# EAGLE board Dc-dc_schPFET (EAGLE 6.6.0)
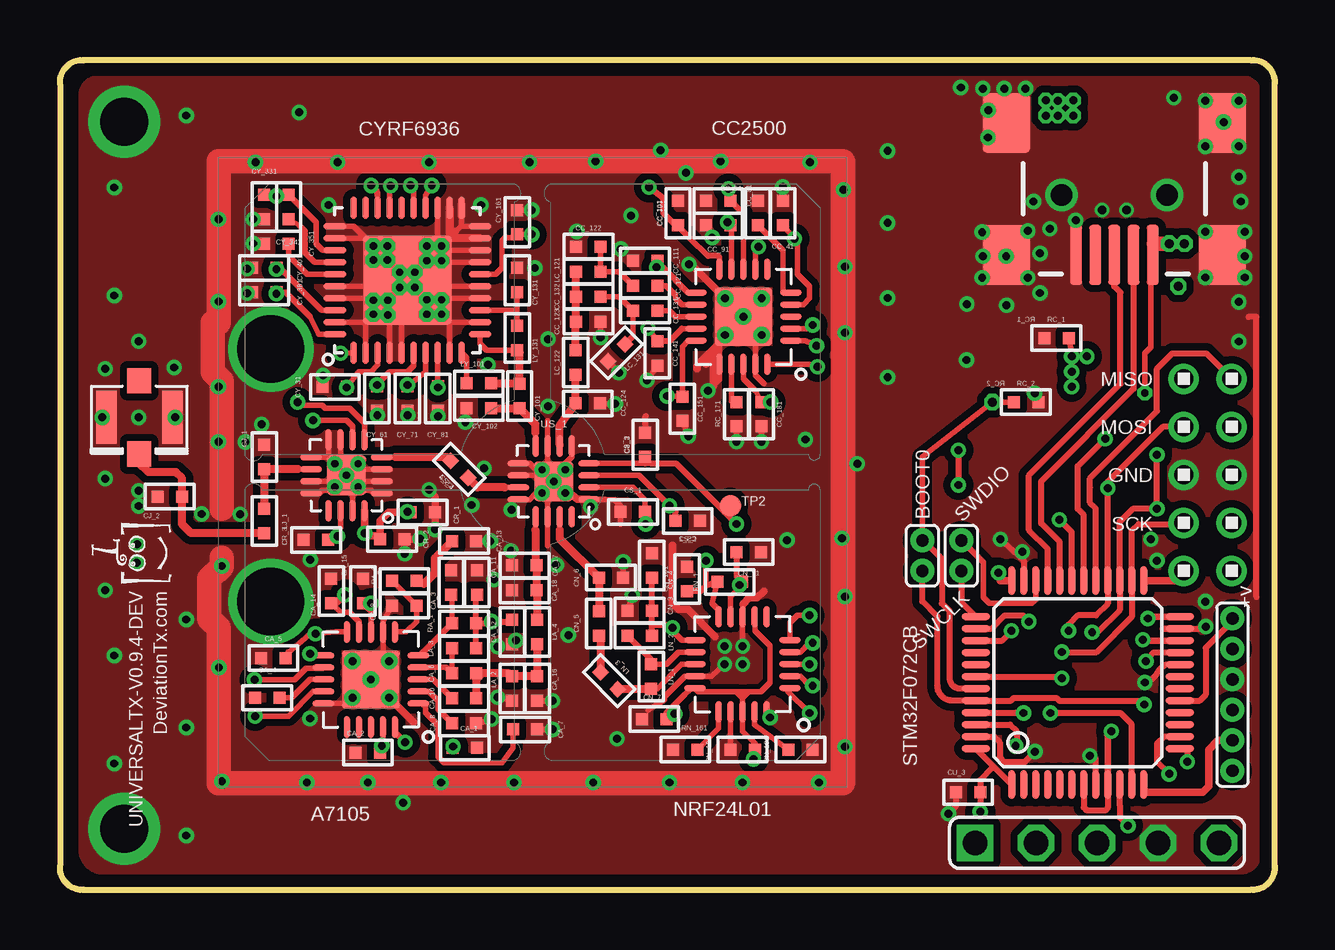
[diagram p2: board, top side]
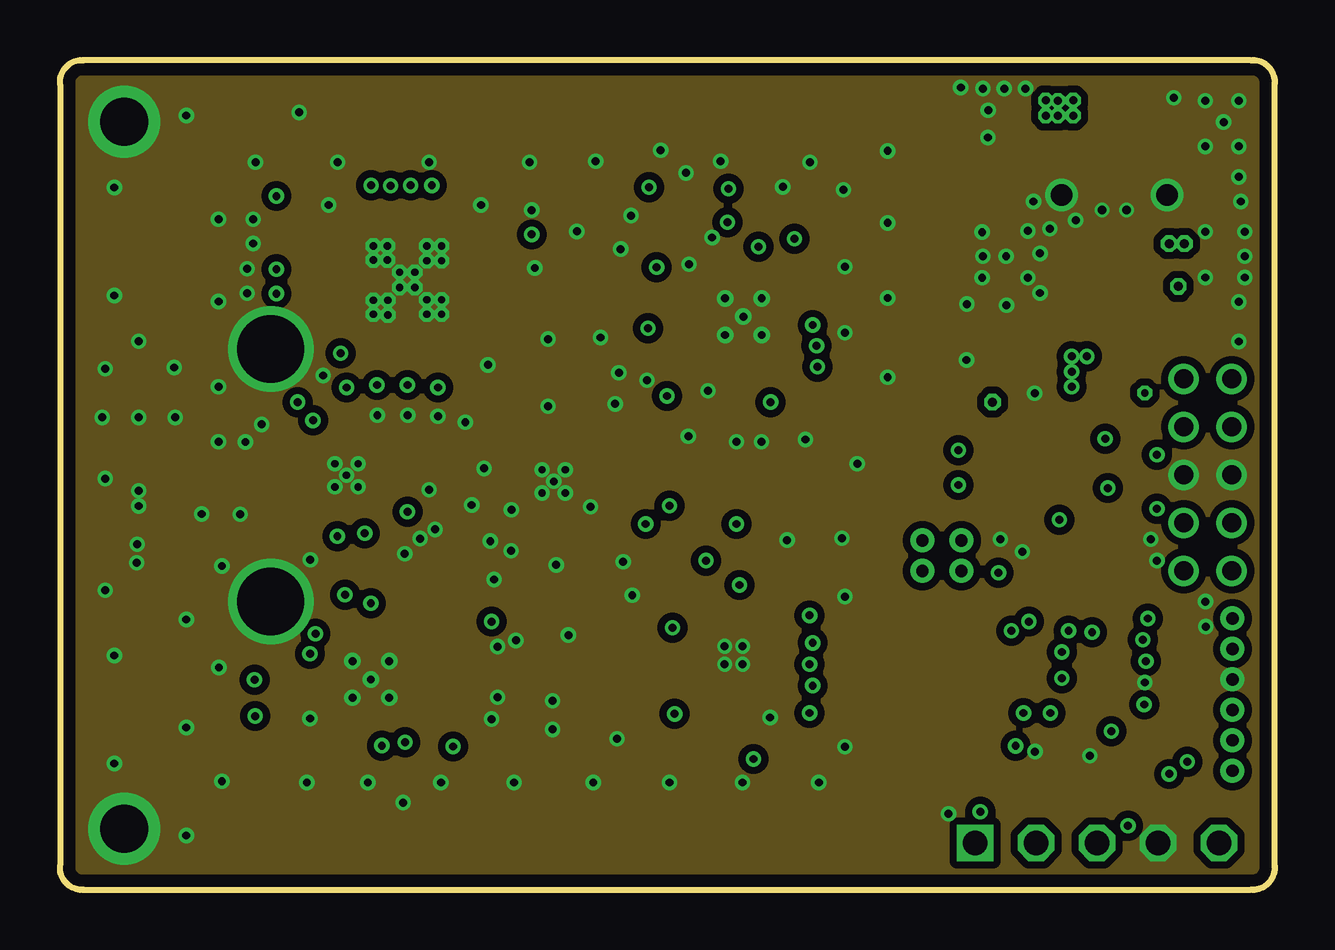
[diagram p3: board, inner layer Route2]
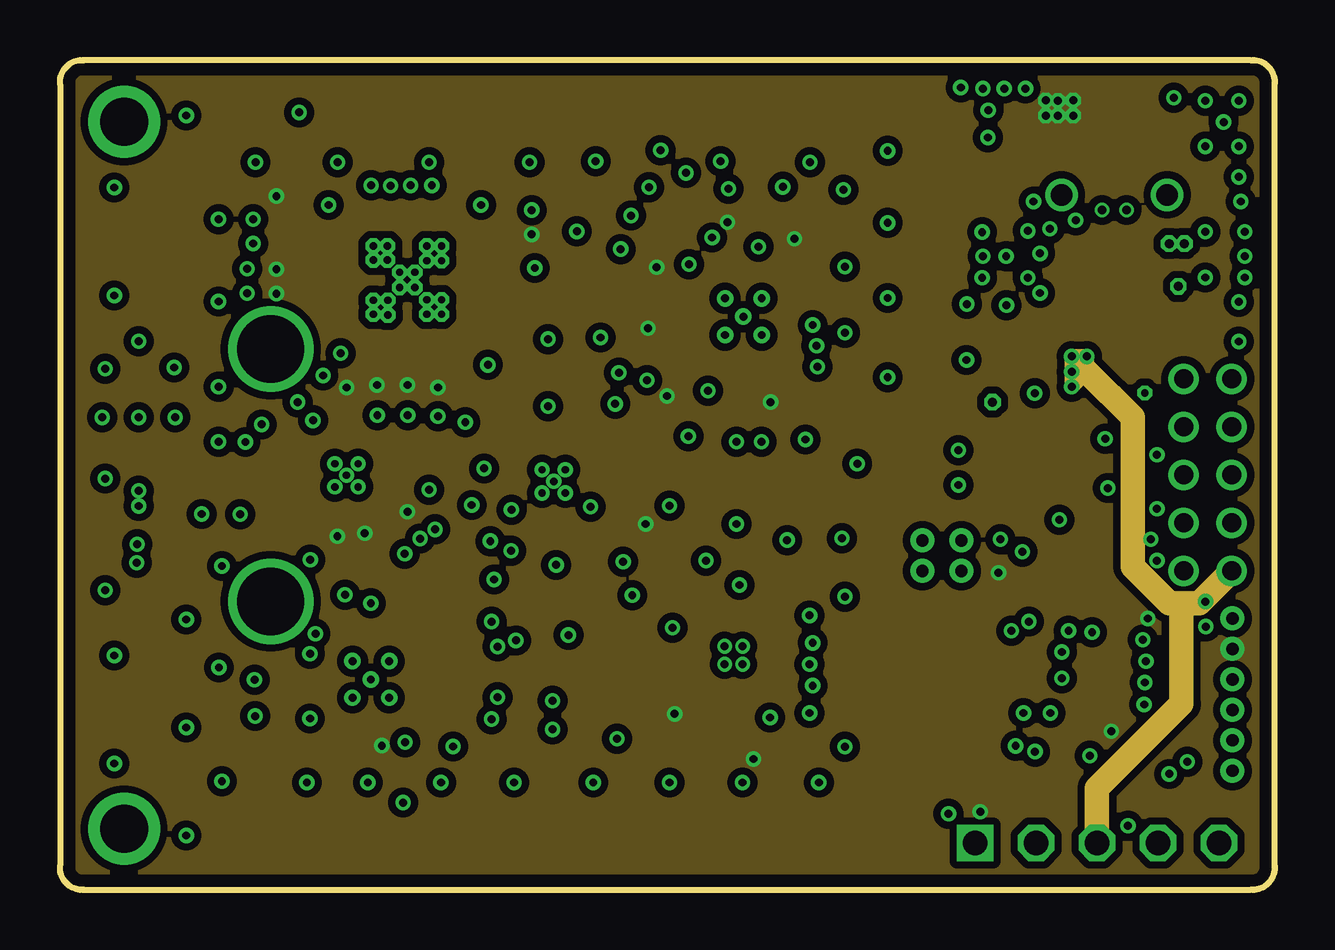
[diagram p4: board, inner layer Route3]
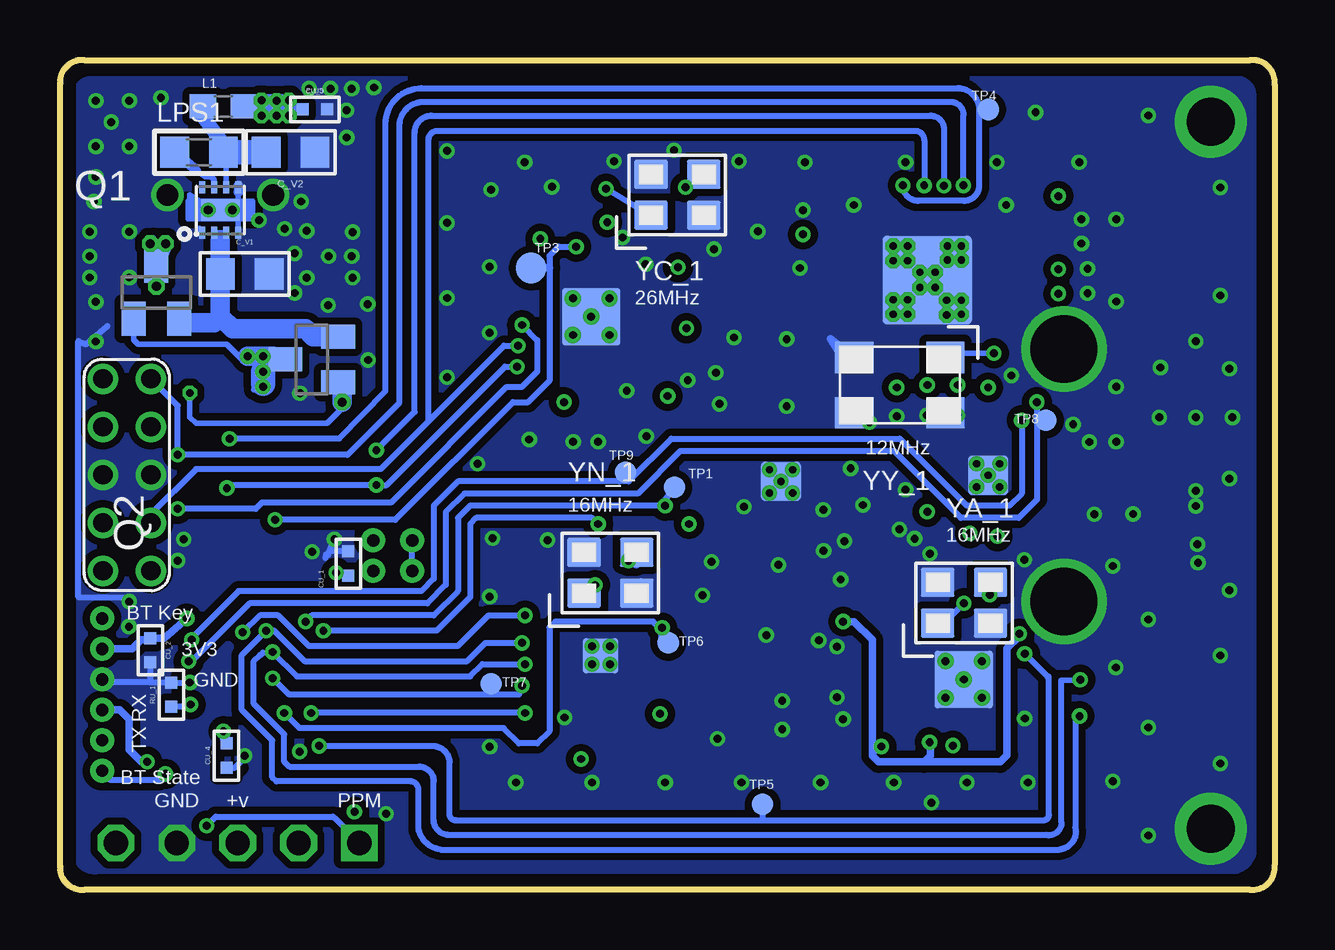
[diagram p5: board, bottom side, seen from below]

Size 50.63 x 34.58 mm. Coordinates in mm from the lower left corner, seen from the top.
Outline: 1.02,0 49.61,0 arc102 50.63,1.02 50.63,33.56 arc102 49.61,34.57 1.02,34.57 arc102 0,33.56 0,1.02 arc102 1.02,0
Copper layers (1*2*3*16): Top 0.035mm / dielectric 1.5mm / Route2 0.035mm / dielectric 0.15mm / Route3 0.035mm / dielectric 0.2mm / Bottom 0.035mm
Design rules "Smart-P-EagleRules *": minimum track width 9mil, minimum drill 12mil, track to track 8mil, track to pad 7mil, pad to pad 7mil, via to via 7mil, smd to smd 0mil, copper to edge 20mil, drill to drill 10mil, minimum pad ring 1mil, minimum via ring 6mil, stop-mask expansion 2mil, vias tented up to drill 25mil, thermal gap 10mil
bRestrict: 9 lines

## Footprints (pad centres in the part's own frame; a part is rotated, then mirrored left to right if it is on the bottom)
PH005-1-2 = drill 0.508 pad 1: 1 0,0; 2 1.27,0
C0805 = smd 1.2 x 1.3: 1 -1.016,0; 2 1.016,0
C0402 = smd 0.5 x 0.5: 1 -0.508,0; 2 0.508,0
LQFP48 = smd 0.3 x 1.2: 1 -2.75,-4.25; 2 -2.25,-4.25; 3 -1.75,-4.25; 4 -1.25,-4.25; 5 -0.75,-4.25; 6 -0.25,-4.25; 7 0.25,-4.25; 8 0.75,-4.25; 9 1.25,-4.25; 10 1.75,-4.25; 11 2.25,-4.25; 12 2.75,-4.25; 25 2.75,4.25; 26 2.25,4.25; 27 1.75,4.25; 28 1.25,4.25; 29 0.75,4.25; 30 0.25,4.25; 31 -0.25,4.25; 32 -0.75,4.25; 33 -1.25,4.25; 34 -1.75,4.25; 35 -2.25,4.25; 36 -2.75,4.25 | smd 1.2 x 0.3: 13 4.25,-2.75; 14 4.25,-2.25; 15 4.25,-1.75; 16 4.25,-1.25; 17 4.25,-0.75; 18 4.25,-0.25; 19 4.25,0.25; 20 4.25,0.75; 21 4.25,1.25; 22 4.25,1.75; 23 4.25,2.25; 24 4.25,2.75; 37 -4.25,2.75; 38 -4.25,2.25; 39 -4.25,1.75; 40 -4.25,1.25; 41 -4.25,0.75; 42 -4.25,0.25; 43 -4.25,-0.25; 44 -4.25,-0.75; 45 -4.25,-1.25; 46 -4.25,-1.75; 47 -4.25,-2.25; 48 -4.25,-2.75
U.FL = smd 2.2 x 0.85: P$1 0,1.375; P$2 0,-1.375 | smd 1.05 x 1: P$3 1.525,0; P$4 -1.525,0
2X5 = drill 0.8 pad 1.27: 1 -4,-1; 2 -4,1; 3 -2,-1; 4 -2,1; 5 0,-1; 6 0,1; 7 2,-1; 8 2,1; 9 4,-1; 10 4,1
1X05-S = drill 1.016 square: 1 -5.08,0 | drill 1.016 octagon: 2 -2.54,0; 3 0,0; 4 2.54,0; 5 5.08,0
PH005-1-6 = drill 0.508 pad 1: 1 0,0; 2 1.27,0; 3 2.54,0; 4 3.81,0; 5 5.08,0; 6 6.35,0
USB-MINIB = drill 0.9 pad 1.016: . 0,2.2; .. 0,-2.2 | smd 2.5 x 0.5: D+ 2.5,0; D- 2.5,0.8; GND 2.5,-1.6; ID 2.5,-0.8; VBUS 2.5,1.6 | smd 2.5 x 2: MTN1 -3,4.5; MTN2 2.5,4.5; MTN3 -3,-4.5; MTN4 2.5,-4.5
0603 = smd 1.1 x 1: 1 -0.85,0; 2 0.85,0
L0402 = smd 0.5 x 0.5: 1 -0.508,0; 2 0.508,0
L0805 = smd 1.2 x 1.3: 1 -1.016,0; 2 1.016,0
WSON-8-PAD = smd 0.25 x 0.5: 1 -0.75,-0.95; 2 -0.25,-0.95; 3 0.25,-0.95; 4 0.75,-0.95; 5 0.75,0.95; 6 0.25,0.95; 7 -0.25,0.95; 8 -0.75,0.95 | drill 0.356 pad 0.61: . -0.508,0; .. 0.508,0 | smd 1.6 x 0.9: PAD 0,0
SOT23 = smd 1 x 1.4: 1 -0.95,-1.1; 2 0.95,-1.1; 3 0,1.1
R0402 = smd 0.5 x 0.5: 1 -0.508,0; 2 0.508,0
TP09R = smd 0.9 x 0.9: TP 0,0
B1,27 = smd 1.27 x 1.27: TP 0,0
1X1 = drill 2: 2 0,0
A7105 = smd 0.9 x 0.25: 1 -1.98,1; 2 -1.98,0.5; 3 -1.98,0; 4 -1.98,-0.5; 5 -1.98,-1; 11 1.98,-1; 12 1.98,-0.5; 13 1.98,0; 14 1.98,0.5; 15 1.98,1 | smd 0.25 x 0.9: 6 -1,-1.98; 7 -0.5,-1.98; 8 0,-1.98; 9 0.5,-1.98; 10 1,-1.98; 16 1,1.98; 17 0.5,1.98; 18 0,1.98; 19 -0.5,1.98; 20 -1,1.98 | smd 2.4 x 2.4: 21 0,0 | smd 2.4 x 2.4 bottom: 22 0,0 | drill 0.33 pad 0.686: P$1 -0.762,0.762; P$2 0.762,0.762; P$3 -0.762,-0.762; P$4 0.762,-0.762; P$9 0,0
CC2500 = smd 0.9 x 0.25: 1 -1.98,1; 2 -1.98,0.5; 3 -1.98,0; 4 -1.98,-0.5; 5 -1.98,-1; 11 1.98,-1; 12 1.98,-0.5; 13 1.98,0; 14 1.98,0.5; 15 1.98,1 | smd 0.25 x 0.9: 6 -1,-1.98; 7 -0.5,-1.98; 8 0,-1.98; 9 0.5,-1.98; 10 1,-1.98; 16 1,1.98; 17 0.5,1.98; 18 0,1.98; 19 -0.5,1.98; 20 -1,1.98 | smd 2.4 x 2.4: 21 0,0 | smd 2.4 x 2.4 bottom: 22 0,0 | drill 0.33 pad 0.686: P$1 -0.762,0.762; P$2 0.762,0.762; P$3 -0.762,-0.762; P$4 0.762,-0.762; P$9 0,0
QFN20-4X4-NRF = smd 0.9 x 0.25: 1 -1.98,1; 2 -1.98,0.5; 3 -1.98,0; 4 -1.98,-0.5; 5 -1.98,-1; 11 1.98,-1; 12 1.98,-0.5; 13 1.98,0; 14 1.98,0.5; 15 1.98,1 | smd 0.25 x 0.9: 6 -1,-1.98; 7 -0.5,-1.98; 8 0,-1.98; 9 0.5,-1.98; 10 1,-1.98; 16 1,1.98; 17 0.5,1.98; 18 0,1.98; 19 -0.5,1.98; 20 -1,1.98 | smd 1.474 x 1.474 bottom: P$1 0.356,-0.356 | drill 0.33 pad 0.61: P$5 0,-0.75; P$6 0.75,0; P$7 0.75,-0.75; P$9 0,0
QFN16-3X3-PAD = smd 0.9 x 0.25: 1 -1.475,0.75; 2 -1.475,0.25; 3 -1.475,-0.25; 4 -1.475,-0.75; 9 1.475,-0.75; 10 1.475,-0.25; 11 1.475,0.25; 12 1.475,0.75 | smd 0.25 x 0.9: 5 -0.75,-1.475; 6 -0.25,-1.475; 7 0.25,-1.475; 8 0.75,-1.475; 13 0.75,1.475; 14 0.25,1.475; 15 -0.25,1.475; 16 -0.75,1.475 | smd 1.65 x 1.65: 17 0,0 | smd 1.65 x 1.65 bottom: 18 0,0 | drill 0.305 pad 0.635: P$1 -0.483,0.483; P$2 0.483,0.483; P$3 0.483,-0.483; P$4 -0.483,-0.483; P$5 0,0
CYRF6936 = smd 0.95 x 0.28: 1 -3.025,2.25; 2 -3.025,1.75; 3 -3.025,1.25; 4 -3.025,0.75; 5 -3.025,0.25; 6 -3.025,-0.25; 7 -3.025,-0.75; 8 -3.025,-1.25; 9 -3.025,-1.75; 10 -3.025,-2.25; 21 3.025,-2.25; 22 3.025,-1.75; 23 3.025,-1.25; 24 3.025,-0.75; 25 3.025,-0.25; 26 3.025,0.25; 27 3.025,0.75; 28 3.025,1.25; 29 3.025,1.75; 30 3.025,2.25 | smd 0.28 x 0.95: 11 -2.25,-3.025; 12 -1.75,-3.025; 13 -1.25,-3.025; 14 -0.75,-3.025; 15 -0.25,-3.025; 16 0.25,-3.025; 17 0.75,-3.025; 18 1.25,-3.025; 19 1.75,-3.025; 20 2.25,-3.025; 31 2.25,3.025; 32 1.75,3.025; 33 1.25,3.025; 34 0.75,3.025; 35 0.25,3.025; 36 -0.25,3.025; 37 -0.75,3.025; 38 -1.25,3.025; 39 -1.75,3.025; 40 -2.25,3.025 | smd 3.7 x 3.7: P$1 0,0 | drill 0.305 pad 0.635 octagon: P$2 -0.838,0.813; P$3 -1.448,0.813; P$4 -1.422,1.422; P$5 -0.838,1.422; P$6 0.838,1.422; P$7 1.422,1.422; P$8 1.422,0.838; P$9 0.838,0.838; P$10 -0.305,0.33; P$11 0.33,0.33; P$12 0.33,-0.305; P$13 -0.305,-0.305; P$14 -1.422,-0.813; P$15 -0.813,-0.813; P$16 -0.813,-1.422; P$17 -1.422,-1.422; P$18 0.813,-0.813; P$19 1.422,-0.813; P$20 1.422,-1.422; P$21 0.813,-1.422 | smd 3.7 x 3.7 bottom: P$23 0,0
3.2X2.5MM = smd 1.4 x 1.2: 1 -1.1,-0.85; 2 1.1,-0.85; 3 1.1,0.85; 4 -1.1,0.85
5X3.2MM = smd 1.6 x 1.3: 1 -1.9,-1.15; 2 1.9,-1.15; 3 1.9,1.15; 4 -1.9,1.15

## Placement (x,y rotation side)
1  BOOT0  [PH005-1-2]  35.95,14.56 270 top
C_V1  10uF  [C0805]  42.93,25.66 0 bottom
C_V2  22uF  [C0805]  41.03,30.74 0 bottom
CA_1  2.2uF  [C0402]  16.87,5.92 0 top
CA_2  2.2uF  [C0402]  12.83,5.72 180 top
CA_3  10pF  [C0402]  16.31,12.81 90 top
CA_4  2.2uF  [C0402]  8.64,8.01 180 top
CA_5  0.1uF  [C0402]  8.89,9.66 180 top
CA_6  10pF  [C0402]  16.85,9.02 0 top
CA_7  120pF  [C0402]  19.39,6.69 0 top
CA_8  1.5nF  [C0402]  16.85,6.94 0 top
CA_9  680pF  [C0402]  14.36,11.84 180 top
CA_10  22pF  [C0402]  16.85,7.98 0 top
CA_11  NC  [C0402]  17.38,12.81 90 top
CA_12  100pF  [C0402]  18.85,10.75 270 top
CA_13  10nF  [C0402]  16.85,14.53 0 top
CA_14  9pF  [C0402]  11.31,12.45 90 top
CA_15  9pF  [C0402]  12.63,12.45 90 top
CA_16  1.0pF  [C0402]  19.89,8.39 270 top
CA_17  1.0pF  [C0402]  19.36,13.52 180 top
CA_18  1.0pF  [C0402]  19.36,12.48 180 top
CC_41  0.1uF  [C0402]  30.13,28.2 90 top
CC_51  0.1uF  [C0402]  29.09,28.2 90 top
CC_81  15pF  [C0402]  27.44,28.71 180 top
CC_91  220pF  [C0402]  27.44,27.69 180 top
CC_101  15pF  [C0402]  25.76,28.2 90 top
CC_111  0.1uF  [C0402]  24.39,26.22 180 top
CC_121  100pF  [C0402]  24.39,25.18 180 top
CC_122  1.0pF  [C0402]  22.03,26.8 180 top
CC_123  1.8pF  [C0402]  22.03,23.68 0 top
CC_124  1.5pF  [C0402]  22,20.27 0 top
CC_131  100pF  [C0402]  24.39,24.13 180 top
CC_132  1.0pF  [C0402]  22.03,24.72 180 top
CC_141  0.1uF  [C0402]  24.9,22.36 270 top
CC_151  220pF  [C0402]  25.94,20.05 270 top
CC_181  220pF  [C0402]  29.24,19.82 270 top
CJ_1  2pF  [C0402]  8.51,18.04 90 top
CJ_2  2pF  [C0402]  4.58,16.39 180 top
CN_3  2.2nF  [C0402]  24.16,11.64 180 top
CN_4  4.7pF  [C0402]  24.67,13.52 90 top
CN_5  1.5pF  [C0402]  22.46,11.1 90 top
CN_6  1.0pF  [C0402]  22.97,13.01 0 top
CN_71  1nF  [C0402]  24.77,7.12 180 top
CN_91  15pF  [C0402]  28.71,14.08 0 top
CN_101  15pF  [C0402]  26.14,12.96 90 top
CN_181  10nF  [C0402]  28.45,5.85 180 top
CN_191  33nF  [C0402]  30.87,5.85 0 top
CR_1  2.2uF  [C0402]  15.12,15.73 0 top
CR_2  10nF  [C0402]  13.85,14.61 0 top
CR_3  220pF  [C0402]  10.67,14.58 180 top
CS_1  0.1uF  [C0402]  23.88,15.75 180 top
CS_2  100pF  [C0402]  26.17,15.37 180 top
CS_3  100pF  [C0402]  24.39,18.55 90 top
CS_4  9pF  [C0402]  16.64,17.53 135 top
CU_1  1uF  [C0402]  38.61,13.59 90 bottom
CU_2  0.1uF  [C0402]  46.87,9.99 270 bottom
CU_3  0.1uF  [C0402]  37.85,4.07 180 top
CU_4  0.1uF  [C0402]  43.69,5.59 270 bottom
CU_5  1uF  [C0402]  40.01,32.52 0 bottom
CY_31  47nF  [C0402]  11.46,20.96 180 top
CY_61  47nF  [C0402]  13.21,20.48 90 top
CY_71  47nF  [C0402]  14.48,20.48 270 top
CY_81  47nF  [C0402]  15.75,20.48 270 top
CY_101  15pF  [C0402]  19.16,20.58 270 top
CY_102  1.5pF  [C0402]  17.45,20.07 180 top
CY_131  2pF  [C0402]  19.05,25.4 90 top
CY_161  47nF  [C0402]  19.05,27.82 90 top
CY_331  47nF  [C0402]  8.51,28.45 90 top
CY_341  0.47uF  [C0402]  9.53,28.45 90 top
CY_351  0.47uF  [C0402]  9.02,26.93 0 top
CY_381  47nF  [C0402]  8.51,24.9 0 top
CY_401  47nF  [C0402]  8.51,25.91 180 top
IC1  STM32F072CB  [LQFP48]  42.42,8.64 0 top
J1  U.FL  [U.FL]  3.31,19.69 270 top
JP1  2X5  [2X5]  47.84,17.29 90 top
JP2  [1X05-S]  43.23,1.96 0 top
JP3  [PH005-1-6]  48.87,4.96 90 bottom
JP6  USBSMD  [USB-MINIB]  43.95,28.96 270 top
L1  2.2uH  [0603]  43.82,32.64 0 bottom
LA_2  4.7nH  [L0402]  18.85,8.39 270 top
LA_3  1.2nH  [L0402]  16.85,10.06 0 top
LA_4  3.1nH  [L0402]  19.89,10.75 270 top
LC_121  1.2nH  [L0402]  22.03,25.76 0 top
LC_122  1.2nH  [L0402]  21.49,21.98 90 top
LC_131  1.2nH  [L0402]  23.2,22.38 45 top
LJ_1  1.5nH  [L0402]  8.51,15.37 90 top
LN_1  8.2nH  [L0402]  24.64,8.89 90 top
LN_2  2.7nH  [L0402]  24.16,10.6 0 top
LN_3  3.9nH  [L0402]  22.89,8.72 315 top
LPS1  2.2uH  [L0805]  44.84,30.74 0 bottom
LY_101  22nH  [L0402]  17.45,21.11 180 top
LY_131  1.8nH  [L0402]  19.05,22.99 90 top
PS1  TPS62172  [WSON-8-PAD]  43.95,28.33 0 bottom
Q1  BSS84  [SOT23]  46.61,24.9 0 bottom
Q2  BSS84  [SOT23]  40.14,22.1 90 bottom
RA_1  NC  [R0402]  16.85,11.1 0 top
RA_2  200  [R0402]  14.36,12.88 180 top
RC_1  100k  [R0402]  41.53,22.99 0 top
RC_2  100k  [R0402]  40.26,20.32 0 top
RC_171  56.2k  [R0402]  28.2,19.82 270 top
RN_1  1M  [R0402]  27.92,12.83 0 top
RN_161  22k  [R0402]  26.07,5.85 180 top
RU_1  47k  [R0402]  45.99,8.13 90 bottom
SWCLK  SWDIO  [PH005-1-2]  37.57,14.56 270 top
TP1  TPTP09R  [TP09R]  25.02,16.77 0 bottom
TP2  TPTP09R  [TP09R]  27.94,16.01 0 top
TP3  TPB1,27  [B1,27]  30.99,25.91 0 bottom
TP4  TPTP09R  [TP09R]  11.94,32.52 0 bottom
TP5  TPTP09R  [TP09R]  21.34,3.56 0 bottom
TP6  TPTP09R  [TP09R]  25.28,10.29 0 bottom
TP7  TPTP09R  [TP09R]  32.66,8.59 0 bottom
TP8  TPTP09R  [TP09R]  9.53,19.56 0 bottom
TP9  TPTP09R  [TP09R]  27.06,17.4 0 bottom
U$1  1X1  [1X1]  2.67,2.54 0 top
U$2  1X1  [1X1]  2.67,32.01 0 top
U$3  SHIELDBMI-S-203  [BMI-S-203-F]  19.69,17.4 0 top
UA_1  A7105  [A7105]  12.96,8.77 180 top
UC_1  CC2500  [CC2500]  28.49,23.88 180 top
UN_1  NRF24L01  [QFN20-4X4-NRF]  28.45,9.4 180 top
UNIVERSALTX-V0.9.4-DEV  LITTLE-GUYLITTLE-GUY-X  [LITTLE-GUY-X]  4.45,12.45 90 top
UR_1  RFX2401C  [QFN16-3X3-PAD]  11.94,17.28 180 top
US_1  PE42641  [QFN16-3X3-PAD]  20.58,17.02 180 top
UY_1  CYRF6936  [CYRF6936]  14.48,25.4 90 top
YA_1  16MHz  [3.2X2.5MM]  12.95,11.96 0 bottom
YC_1  26MHz  [3.2X2.5MM]  24.9,28.96 0 bottom
YN_1  16MHz  [3.2X2.5MM]  27.69,13.21 0 bottom
YY_1  12MHz  [5X3.2MM]  15.63,21.04 180 bottom

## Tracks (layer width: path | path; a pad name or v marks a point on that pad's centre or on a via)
+3V3  (via drill 0.33, 0.33 pad 0.64)
  Top 0.229: UN_1.7 28.96,11.29 28.96,10.8 29.6,10.16 29.6,8.64 29.21,8.26 28.71,8.26 | v29.62,20.32 CC_181.1 28.99,20.81 28.49,21.31 UC_1.18 | UC_1.15 26.18,22.88 25.94,22.64 CC_151.1 25.66,20.58 v25.3,20.58 | CC_111.1 v24.87,25.94 25.13,25.94 26.18,24.88 UC_1.11 | CC_141.1 v24.52,23.4 | UC_1.14 25.92,23.38 | v19.66,27.31 CY_161.1 18.93,27.18 18.55,27.18 18.42,27.06 18.42,25.91 18.16,25.65 UY_1.16 | UY_1.3 13.24,21.87 12.96,21.59 12.45,21.59 CY_31.1 v11.94,20.93 | UY_1.6 14.73,21.84 14.48,21.59 13.75,21.59 13.29,21.14 CY_61.2 13.21,20.93 | UY_1.7 15.23,21.58 CY_71.1 14.48,20.93 | UY_1.33 10.95,26.65 10.67,26.93 10.67,27.82 CY_341.2 | CS_1.1 24.39,16.26 23.88,16.77 US_1.2 | CC_41.1 v30.61,27.13 30.74,26.95 30.74,25.66 31.25,25.15 31.25,24.64 30.99,24.38 UC_1.4 | 28.71,8.26 28.45,8.01 | 28.45,8.01 28.2,8.26 | 28.2,8.26 26.62,8.26 UN_1.15 | 28.45,8.01 UN_1.18 28.45,6.61 28.96,6.1 CN_181.1 28.96,5.5 v28.91,5.45 | 28.2,8.26 28.71,8.26 | UY_1.38 10.91,24.15 9.15,25.91 CY_401.1 v9.02,25.86 | UY_1.40 10.79,23.15 10.43,23.88 9.4,24.9 CY_381.2 v9.02,24.85 | v15.75,20.93 CY_81.1 15.73,21 UY_1.8 | 12.69,14.75 12.69,14.85 v12.7,14.86 | UR_1.14 11.69,15.1 CR_3.1 11.41,14.58 v11.56,14.74 | UA_1.19 13.46,6.22 | v25.62,7.33 25.48,7.57 26.04,8.13 26.29,8.39 | UC_1.9 27.99,27.65 CC_91.1 v27.82,27.82
  Top 0.254: IC1.48 IC1.1 38.98,5.08 38.87,5.08 38.36,4.58 CU_3.1 v38.36,3.26 | 25.92,23.38 25.4,22.86 CC_141.1 | IC1.7 42.67,3.44 42.8,3.31 43.57,3.31 43.67,3.41 IC1.9 | CY_61.2 v13.21,21.04 | v14.48,21.04 CY_71.1 | CS_1.1 24.41,15.73 v24.41,15.24 | 26.04,8.13 25.28,7.37 CN_71.1
  Top 0.279: IC1.24 45.51,11.39 | IC1.9 43.67,6.46
  Top 0.305: 43.67,6.46 v43.82,6.61 | 45.51,11.39 v45.34,11.31 | IC1.36 39.19,12.89 v39.12,13.21 | UR_1.16 12.69,14.75 | 12.69,14.75 12.7,14.74 | 12.69,14.75 13.2,14.75 CR_2.1 13.34,15.37 13.7,15.73 CR_1.1 | 8.46,28.91 CY_331.2 8.97,28.96 v9.02,28.91 9.07,28.96 CY_341.2 | 13.46,6.22 13.46,6.05 v13.42,6.01 13.34,5.94 CA_2.1
  Bottom 0.229: 41.41,32.64 v41.09,32.9
  Bottom 0.254: CU_1.1 v39.12,13.21 | CU_2.1 46.87,10.44 46.89,10.42
  Bottom 0.305: CU_2.1 46.28,10.49 v45.34,11.31 | JP3.5 47.63,10.04 47.25,10.42 46.89,10.42 46.74,10.42
  Bottom 0.406: CU_4.1 v43.82,6.61 | CU_5.1 42.11,32.39 v42.23,32.26
  Bottom 1.016: L1.2 41.41,32.64
  other vias: 14.48,15.75 41.6,32.89 41.6,32.26 41.09,32.26 42.23,32.9
  pour Route3 (isolate 0.305, no thermals): 0.56,34.23 0.56,0.56 50.23,0.56 50.23,34.23
+5V  (via drill 0.33 pad 0.64)
  Top 0.229: RC_1.2 42.17,22.36 v42.17,22.23 v42.17,20.96
  Route3 0.61: v42.8,22.23 42.8,21.59 v42.17,20.96 v42.17,21.59 v42.17,22.23 v42.8,22.23
  Route3 1.016: JP1.1 47.49,11.94 46.74,11.94 | 46.74,11.94 46.23,11.94 44.71,13.47 44.71,19.69 42.8,21.59 | 46.74,11.94 46.74,7.75 43.23,4.24 JP2.3
  Bottom 0.229: 42.55,20.83 v42.17,20.96 | Q1.1 47.56,22.93 47.38,22.74 43.69,22.74 43.06,22.1 42.93,22.1 v42.8,22.23
  Bottom 0.305: 42.17,22.1 v42.17,22.23 42.42,22.23 42.42,21.09 42.17,21.09
  Bottom 0.813: Q2.3 41.74,22.23 v42.8,22.23
  Bottom 1.016: 42.17,21.09 v42.17,21.59
A7105_CSN  (via drill 0.33, 0.33 pad 0.64)
  Top 0.229: UA_1.11 10.49,9.77 v10.42,9.84
  Top 0.254: IC1.46 39.6,6.89 39.88,6.61 39.88,5.97 v39.83,6
  Bottom 0.254: 21.34,2.9 34.09,2.9 arc108 34.4,3.2 34.4,5.29 arc-90 35.11,6 v39.83,6 | 21.34,2.9 9.63,2.9 arc-108 9.43,3.18 9.43,8.9 9.48,8.9 v10.42,9.84 | TP5.TP 21.34,2.9
BT_KEY
  Top 0.254: IC1.17 47.51,7.89 47.76,8.13 47.76,10.09 48.9,11.23 48.9,11.28 JP3.6
BT_STATE  (via drill 0.33)
  Top 0.254: IC1.14 46.01,6.39 45.72,6.1 45.72,5.34 v46.23,4.83
  Bottom 0.254: v46.23,4.83 46.49,4.58 48.52,4.58 48.87,4.93 JP3.1
CC_CSN  (via drill 0.33)
  Top 0.229: UC_1.7 28.99,26.68 v29.11,26.8
  Top 0.254: IC1.31 42.17,14.91 v41.66,15.42
  Bottom 0.254: v41.66,15.42 36.66,15.42 31.75,20.32 31.12,20.32 30.23,21.21 30.23,25.91 30.23,26.42 29.85,26.8 v29.11,26.8
  Bottom 0.305: TP3.TP 30.23,25.91
CYRF_CSN  (via drill 0.33)
  Top 0.229: UY_1.24 15.23,28.95 v15.5,29.35
  Top 0.254: IC1.30 42.67,15.63 42.42,15.88 42.42,17.66 v43.57,18.8
  Bottom 0.254: v43.57,18.8 38.99,18.8 37.06,20.78 37.06,31.91 arc90 35.56,33.41 13.21,33.41 arc90 12.32,32.52 | 12.32,32.52 12.32,29.34 arc90 12.96,28.71 14.85,28.71 arc90 v15.5,29.35 | TP4.TP 12.32,32.52
LINK  (via drill 0.33 pad 0.64)
  Top 0.254: 1.2 35.95,12.02 36.58,11.38 36.58,8.51 arc92 37.2,7.89 IC1.44 39.64,7.89 39.76,8.01 41.53,8.01 41.66,7.88 44.96,7.88 v45.19,7.73
  Bottom 0.254: v45.19,7.73 45.29,7.62 RU_1.1
MISO  (via drill 0.33, 0.33 pad 0.64)
  Top 0.229: UY_1.28 13.23,28.94 | UC_1.2 31.21,23.38 v31.37,23.54 | UN_1.5 30.43,11.13 30.74,11.43 v31.25,11.43
  Top 0.254: v45.72,18.13 v45.72,15.88 44.71,15.88 44.17,15.34 IC1.27 44.17,11.66 43.25,10.74 v43.02,10.74 | 13.23,28.94 13.23,28.99 arc45 13.16,29.17 v12.97,29.35
  Bottom 0.254: v45.72,18.13 45.72,20.17 JP1.10 | 45.69,18.04 v45.72,18.13 | v45.72,15.88 42.47,15.88 42.22,16.13 36.83,16.13 32.01,20.96 31.37,20.96 30.74,21.59 30.74,22.9 v31.37,23.54 | v45.72,18.13 38.65,18.13 36.48,20.3 36.48,31.86 arc90 35.45,32.83 13.51,32.83 arc90 12.97,32.3 v12.97,29.35 | v43.02,10.74 42.3,11.43 41.53,11.43 40.26,10.16 34.04,10.16 32.77,11.43 v31.25,11.43
MOSI  (via drill 0.33, 0.33 pad 0.64)
  Top 0.229: UN_1.4 30.73,9.9 30.74,9.91 30.87,9.91 31.25,10.29 v31.37,10.29 | UC_1.20 31.22,21.9 v31.58,21.8 | UA_1.14 10.55,8.27 9.53,7.24 v8.13,7.24 | UY_1.27 13.73,29.22 arc-45 v13.78,29.34
  Top 0.254: v43.67,16.74 IC1.28 43.67,11.92 43.18,11.43 42.42,11.43 42.04,11.05 v42.04,10.8 | v43.67,16.74 43.68,16.62 | v37.44,18.32 v37.44,16.87 | v43.67,16.74 43.67,16.88 | JP1.8 45.96,19.29 43.67,17 v43.67,16.74
  Bottom 0.254: v43.67,16.74 43.67,16.79 43.44,16.87 v37.44,16.87 37.01,16.87 32.08,21.8 v31.58,21.8 | v37.44,18.32 35.84,19.92 35.84,31.55 arc90 35.13,32.26 14.36,32.26 arc90 13.78,31.69 v13.78,29.34 | v8.13,7.24 8.31,7.17 8.31,2.6 arc96 8.97,1.68 34.78,1.68 arc75 35.69,2.6 35.69,4.22 arc-75 36,4.53 41.61,4.53 41.79,4.7 41.79,6.23 43.06,7.5 43.06,9.78 v42.04,10.8 41.71,10.8 40.44,9.53 33.66,9.53 32.9,10.29 v31.37,10.29
MUXSEL1  (via drill 0.33)
  Top 0.229: 24.14,17.27 US_1.3
  Top 0.254: 24.14,17.27 v25.4,16.01 25.66,15.75 CS_2.2 | IC1.38 38.83,10.89 39.37,11.43 40.14,11.43 v40.39,11.18
  Bottom 0.254: v40.39,11.18 40.14,11.43 35.06,11.43 34.04,12.45 34.04,15.5 33.53,16.01 v25.4,16.01 25.4,16.26 TP1.TP
MUXSEL2  (via drill 0.33, 0.33 pad 0.64)
  Top 0.229: US_1.4 24.39,17.77 24.65,17.77 | TP2.TP 27.69,15.75
  Top 0.254: IC1.39 39.27,10.39 v39.65,10.8 | CS_3.1 24.39,17.77 | 24.65,17.77 25.67,17.77 27.69,15.75 v28.2,15.24
  Bottom 0.254: v39.65,10.8 34.93,10.8 33.53,12.2 33.53,15.24 33.28,15.5 28.45,15.5 v28.2,15.24
N$1  (via drill 0.33 pad 0.64)
  Top 0.229: UN_1.10 27.45,11.67 27.18,11.94 RN_1.1
  Top 0.254: RN_1.1 26.93,12.68 | 26.93,12.68 v26.93,13.72 | 26.93,12.68 26.7,12.45 CN_101.1
  Bottom 0.254: 26.25,13.72 YN_1.3 26.59,13.51 v26.93,13.72
N$2  (via drill 0.33 pad 0.64)
  Top 0.229: UN_1.9 27.95,12.2 28.33,12.58 v28.33,12.7 28.33,12.73 RN_1.2
  Top 0.254: CN_91.1 28.2,13.06 RN_1.2
  Bottom 0.254: YN_1.1 28.96,12.53 v28.33,12.7
N$3
  Top 0.229: UN_1.19 28.95,6.87 CN_191.1
N$4
  Top 0.229: RA_2.2 CA_9.1 14.86,11.18 14.43,10.75 UA_1.6
N$5
  Top 0.229: UN_1.13 25.91,9.4 24.9,8.39 LN_1.1 | 23.28,8.39 LN_3.2
  Top 0.33: 23.28,8.39 LN_1.1
N$7
  Top 0.33: LJ_1.1 5.47,14.86 5.08,15.24 CJ_2.1 5.08,17.15 4.83,17.4 3.69,17.4 3.31,17.78 J1.P$3
N$8
  Top 0.229: 22.46,9.15 LN_3.1
  Top 0.33: CN_5.1 22.53,10.52 LN_3.1
N$9
  Top 0.229: US_1.15 20.83,15.12 20.83,14.99
  Top 0.33: 20.83,14.99 20.83,14.63 CN_6.1 CN_5.2
N$10
  Top 0.229: UN_1.16 27.45,6.73 RN_161.1
N$11
  Top 0.254: CA_13.1 16.21,14.41
  Top 0.33: RA_2.1 15.17,12.76 15.63,13.21 15.63,13.82 CA_13.1
N$12  (via drill 0.33)
  Top 0.229: UA_1.9 12.46,11.17 12.07,11.56 11.69,11.56 CA_14.1 11.52,11.94 v11.88,12.3
  Bottom 0.229: YA_1.3 11.85,12.86
  Bottom 0.254: YA_1.3 11.85,13.24 v11.88,12.3
N$14
  Top 0.229: UC_1.13 26.67,23.88 25.66,23.88 25.4,24.13 CC_131.1
N$15
  Top 0.229: UN_1.12 25.78,9.9 25.28,9.4 LN_1.2 24.64,9.61 LN_2.1
N$16
  Top 0.229: UC_1.12 25.92,24.38 25.66,24.64 25.66,24.77 25.25,25.18 CC_121.1
N$17  (via drill 0.33)
  Top 0.229: UA_1.8 12.96,11.61 CA_15.1 v12.96,11.94
  Bottom 0.229: 13.79,10.86 YA_1.1 13.79,11.11 v12.96,11.94
N$18
  Top 0.229: UA_1.13 10.42,8.77 9.66,8.01 CA_4.1
N$24
  Top 0.33: LC_122.2 21.49,23.65 CC_123.1 CC_132.2 LC_121.1
N$25
  Top 0.229: 19.83,13.48 CA_17.1 19.83,13.56 | 19.89,12.45 CA_18.1 19.84,12.5 | US_1.13 19.83,15.13 19.82,14.99
  Top 0.33: 19.82,14.99 19.82,13.57 CA_17.1 CA_18.1 | 19.89,12.45 LA_4.1
N$26
  Top 0.229: CA_7.1 18.88,5.92 18.42,5.29 16.01,5.29 15.75,5.54 15.75,6.86 15.24,7.37 15.24,7.62 15.1,7.77 UA_1.1
N$27
  Top 0.229: UA_1.2 15.36,8.27 15.75,7.88 15.75,7.52 CA_8.1
N$28
  Top 0.229: UA_1.3 15.55,8.77 CA_10.1
N$29
  Top 0.229: 16.22,9.01 CA_6.1 | LA_3.1 CA_6.1 | UA_1.4 16.09,9.27 CA_6.1
N$30
  Top 0.229: RA_1.1 16.34,12.27 CA_3.1 | UA_1.5 15.1,9.77 15.1,9.89
  Top 0.254: RA_1.1 15.13,9.89 15.1,9.89
N$31
  Top 0.229: 8.89,17.53 CJ_1.1 | UR_1.10 9.91,17.53
  Top 0.33: 9.91,17.53 CJ_1.1 LJ_1.2
N$32
  Top 0.229: UC_1.5 30.13,24.91 30.13,26.65 CC_51.1
N$33
  Top 0.229: UY_1.35 10.3,25.65 9.53,26.42 CY_351.2
N$34
  Top 0.229: US_1.11 18.55,16.77
  Top 0.33: 18.55,16.77 17.4,16.77 CS_4.1
N$35
  Top 0.229: UR_1.4 13.84,18.03 13.97,18.04
  Top 0.33: 13.97,18.04 16.13,18.04 CS_4.2
N$36
  Bottom 0.229: PS1.7 44.2,29.59 44.33,29.72 44.58,29.72 44.96,29.98
  Bottom 0.406: 44.96,29.98 LPS1.1
N$37
  Top 0.229: UC_1.17 27.99,20.37 RC_171.1
N$38  (via drill 0.33)
  Top 0.229: UC_1.10 27.49,26.37 27.44,26.42
  Top 0.254: 27.44,26.42 27.02,26.42 26.28,27.13 25.76,27.65 CC_101.1 25.66,27.69 25.15,28.2 25.15,28.81 v24.55,29.28
  Bottom 0.254: YC_1.3 23.8,29.63 arc45 23.87,29.45 v24.55,29.28
N$39  (via drill 0.33)
  Top 0.229: UC_1.8 28.49,28.16 CC_81.1
  Top 0.254: v27.87,29.21 27.94,29.14 CC_81.1
  Bottom 0.254: 25.74,28.54 YC_1.1 26.05,28.11 v27.87,29.21
N$40
  Top 0.229: CC_122.1 LC_121.2 23.3,25.76 CC_121.2
N$41
  Top 0.229: LC_131.2 23.88,23.07 CC_131.2 23.3,24.72 CC_132.1
N$42
  Bottom 0.254: 35.95,13.34 35.95,14.48
N$43
  Top 0.229: CY_341.1 9.96,27.69 10.22,27.44 10.22,26.55 10.61,26.15 UY_1.34
N$44  (via drill 0.33 pad 0.64)
  Top 0.229: v11.7,22.36 UY_1.1
  Bottom 0.229: v11.7,22.36 13.62,22.36 YY_1.1
N$45
  Top 0.229: UY_1.10 16.95,22.17 LY_101.2
N$46
  Top 0.229: UY_1.11 17.51,22.76 17.78,22.48 LY_131.1
  Top 0.33: LY_101.1 19.13,21.11 CY_101.1 19.16,22.38 LY_131.1
N$47
  Top 0.229: LY_131.2 CY_131.1 19.03,24.15 UY_1.13
N$48
  Top 0.229: 17.48,8.89 CA_6.2
  Top 0.33: LA_4.2 CA_16.1 LA_2.1 18.72,9.02 CA_6.2 | 17.48,8.89 17.35,8.77 CA_10.2
N$49
  Top 0.229: US_1.8 19.83,19.04 19.82,19.05
  Top 0.33: CY_102.1 CY_101.2 19.82,19.41 19.82,19.05
N$50
  Top 0.229: US_1.6 20.83,18.54 20.83,18.55
  Top 0.33: 20.83,18.55 20.83,19.36 CC_124.1 LC_122.1
N$51
  Bottom 0.229: PS1.6 43.7,30.23 LPS1.2 | 44.71,32.39 44.71,32.6 L1.1
  Bottom 0.61: LPS1.2 43.82,31.12 44.71,32.26 44.71,32.39
  Bottom 1.016: C_V2.1 LPS1.2
NRF_CE  (via drill 0.33)
  Top 0.229: UN_1.1 30.35,8.26 v31.25,7.37
  Top 0.254: IC1.45 39.86,7.39 v40.16,7.37
  Bottom 0.254: v31.25,7.37 v40.16,7.37
NRF_CSN  (via drill 0.33)
  Top 0.229: UN_1.2 30.86,8.9 31.25,8.51 v31.37,8.51
  Top 0.254: IC1.42 41.69,8.89 v41.76,8.82
  Bottom 0.229: 31.5,8.13 v31.37,8.51 | TP7.TP 32.66,8.25 32.77,8.13
  Bottom 0.254: 31.5,8.13 32.77,8.13 41.08,8.13 v41.76,8.82
NRF_PAEN  (via drill 0.33)
  Top 0.229: UN_1.11 25.93,10.4 25.66,10.67 v25.53,10.93
  Top 0.254: CN_4.1 CN_3.1 24.67,11.05 | LN_2.2 24.67,11.05 | v41.28,7.37 44.2,7.37 44.67,6.9 IC1.11 | 24.67,11.05 25.4,11.05 v25.53,10.93
  Bottom 0.254: v25.53,10.93 25.66,10.93 25.91,11.18 29.98,11.18 30.23,10.93 30.23,6.61 30.74,6.1 31.5,6.1 32.14,6.74 40.64,6.74 v41.28,7.37 41.28,7.24
  Bottom 0.305: TP6.TP 25.53,10.55 v25.53,10.93
PPM  (via drill 0.33)
  Top 0.254: IC1.10 44.17,3.53 44.17,3.02 v44.52,2.67
  Bottom 0.254: v44.52,2.67 44.14,3.05 39.25,3.05 39.12,2.94 JP2.1
RF_CSN
  Top 0.305: IC1.25 46.44,12.89 JP1.2
RX_EN  (via drill 0.33, 0.33 pad 0.64)
  Top 0.229: UR_1.6 12.19,19.31 11.94,19.56 v10.55,19.56
  Top 0.254: 45.12,10.39 v45.14,10.42
  Top 0.279: IC1.22 45.12,10.39
  Bottom 0.229: TP9.TP 27.06,17.28 27.31,17.02
  Bottom 0.254: v45.14,10.42 45.14,10.49 43.18,12.45 35.56,12.45 35.06,12.96 35.06,16.01 34.04,17.02 27.31,17.02 26.93,17.02 25.15,18.8 15.63,18.8 12.83,16.01 11.05,16.01 10.55,16.51 v10.55,19.56
SCK  (via drill 0.33, 0.33 pad 0.64)
  Top 0.229: UY_1.25 14.73,29.48 | UN_1.3 v31.25,9.4 | UC_1.1 31.08,22.88 v31.54,22.67 | v8.11,8.75 9.77,8.75 10.25,9.22 10.95,9.22 UA_1.12
  Top 0.254: 14.73,29.48 v14.61,29.35 | JP1.4 46.79,15.24 44.96,15.24 44.67,14.95 IC1.26 44.67,11.37 43.21,9.91 v41.76,9.91 | UC_1.1
  Bottom 0.254: 35.27,19.52 37.27,17.53 44.96,17.53 46.84,15.65 JP1.4 | 35.27,19.52 35.27,31.25 arc90 34.89,31.63 14.99,31.63 arc90 14.61,31.25 v14.61,29.35 | 41.91,9.91 v41.76,9.91 | v41.76,9.91 42.17,9.89 42.3,9.78 42.55,9.53 42.55,7.75 41.28,6.48 41.28,5.34 41.08,5.14 35.67,5.14 arc90 35.06,4.53 35.06,2.9 arc-85 34.45,2.29 9.55,2.29 arc-105 8.88,2.81 8.89,2.82 8.89,8.73 v8.11,8.75 | v41.76,9.91 40.75,8.89 33.53,8.89 33.02,9.4 v31.25,9.4 | 35.27,19.52 32.12,22.67 v31.54,22.67
SWCLK
  Top 0.254: SWCLK.2 37.57,11.99 IC1.37
SWDIO
  Top 0.229: IC1.34 40.67,12.1 40.52,11.94 38.74,11.94 38.49,12.2 38.49,13.64 SWCLK.1
TX_EN  (via drill 0.33, 0.33 pad 0.64)
  Top 0.229: UR_1.5 12.69,19.45 12.07,20.07 11.05,20.07 10.93,20.2 10.04,20.2 v9.91,20.32
  Top 0.254: IC1.21 45.58,9.89 v45.27,9.53
  Bottom 0.254: v45.27,9.53 45.14,9.53 42.73,11.94 35.31,11.94 34.55,12.7 34.55,15.75 33.79,16.51 26.55,16.51 24.77,18.29 15.88,18.29 13.09,15.5 10.67,15.5 9.91,16.26 9.91,19.56 | v9.91,20.32 9.91,19.56 | TP8.TP 9.91,19.56
UART_RX  (via drill 0.33)
  Top 0.254: IC1.13 46.99,5.89 v46.99,5.34
  Bottom 0.305: JP3.3 48.14,7.5 47.76,7.12 47.76,5.85 47.25,5.34 v46.99,5.34
UART_TX
  Top 0.279: IC1.12 45.17,4.07
  Top 0.305: JP3.2 48.27,6.23 47.88,5.85 47.88,4.32 47.63,4.07 45.17,4.07
UC_CSN
  Top 0.254: JP1.9 47.78,22.36 46.36,22.36 45.72,21.72 45.72,19.94 42.93,17.15 42.93,16.77 42.93,16.13 43.17,15.89 IC1.29
USB_D+
  Top 0.254: JP6.D+ 43.95,25.15 44.2,24.9 44.2,21.09 40.39,17.28 40.39,14.99 41.17,14.21 IC1.33
USB_D-
  Top 0.254: JP6.D- 44.75,20.87 40.9,17.02 40.9,16.51 40.9,15.27 41.67,14.5 IC1.32
VBUS  (via drill 0.3 pad 0.41, 0.38)
  Top 0.229: JP6.VBUS 45.47,26.38 45.47,22.61 45.22,22.36 v45.22,20.71 45.22,20.58 | 1.1 35.95,18.04 v38.87,20.32 RC_2.1
  Top 0.254: IC1.43 37.47,8.39 arc-74 37.09,8.77 37.09,11.61 36.76,11.94 36.76,13.8 36,14.56 1.1
  Top 0.305: 45.6,26.93 45.6,26.51 JP6.VBUS
  Top 0.406: v46.23,26.93 v46.87,26.93
  Top 0.61: v46.23,26.93 45.6,26.93
  Bottom 0.229: v46.87,26.93 46.74,27.18 v46.61,25.15 | v38.87,20.32 38.87,20.07 39.5,19.44 44.96,19.44 45.22,19.69 v45.22,20.71
  Bottom 0.61: Q1.3 v46.23,26.93
  Bottom 0.813: Q2.1 38.87,20.98 v38.87,20.32
VIN_LDO
  Bottom 0.229: PS1.3 PS1.2 44.2,27.31 43.95,27.06
  Bottom 0.813: Q2.2 40.07,23.05 40.39,23.37 43.44,23.37 43.95,23.88 | 43.95,23.88 C_V1.1 43.95,27.06 | 43.95,23.88 44.2,23.63 45.49,23.63 Q1.2
VPLL_7105  (via drill 0.33, 0.33 pad 0.64)
  Top 0.229: UA_1.20 13.96,6.57 v14.38,6.15 | UA_1.10 11.48,10.75 v10.65,10.67 | 10.42,10.67 10.08,10.35 9.53,9.91
  Top 0.254: LA_3.2 RA_1.2 | RA_1.2 17.81,11.1 v17.99,11.18 18.78,11.18 CA_12.1 | RA_1.2 17.35,12.27 CA_11.1 | 10.42,10.67 v10.65,10.67 | CA_5.1 9.53,9.91
  Top 0.305: CA_1.1 16.36,5.85 v16.39,5.97
  Bottom 0.305: 14.61,5.34 11.43,5.34 11.16,5.62 11.16,10.06 10.65,10.57 v10.65,10.67 | 14.61,5.34 16.51,5.34 16.77,5.59 | 16.77,5.59 16.77,10.42 17.53,11.18 v17.99,11.18 | 16.77,5.59 arc90 16.44,5.92 CA_1.1 arc90 16.39,5.95 v16.39,5.97 | v14.38,6.15 14.36,5.59 14.61,5.34
VSS  (via drill 0.33, 0.33 pad 0.64, 2.8)
  Top 0.229: CA_17.2 18.8,13.72 v18.8,14.13 | UA_1.7 13.46,9.28 UA_1.P$3 | UR_1.3 12.59,17.53 | 12.59,17.53 12.5,17.7 | UR_1.2 12.59,17.03 UR_1.P$1 | UR_1.11 11.29,17.03 11.29,16.79 11.33,16.79 | UR_1.8 11.19,18.03 | UR_1.15 12.19,16.63 UR_1.P$1 | UR_1.9 11.19,18.03 | 11.19,18.03 UR_1.P$3 11.69,17.99 UR_1.7 | UN_1.P$6 27.15,8.9 UN_1.14 26.05,8.9 25.19,8.04 25.19,7.92 | UN_1.P$5 UN_1.8 28.47,11.9 | 27.73,23.91 27.49,23.91 UC_1.16 27.49,21.26 27.06,20.83 | UC_1.P$1 28.99,23.04 UC_1.19 28.99,21.44 29.34,21.09 | RC_171.2 v28.2,18.67 | CC_181.2 v29.24,18.67 | CY_161.2 v19.66,28.33 | CY_81.2 v15.75,19.74 | 22.74,16.26 23.12,16.26 23.37,16.01 CS_1.2 23.37,15.24 | 22.74,16.26 22.25,16.26 | UY_1.P$18 14.48,26.29 UY_1.P$12 | 13.47,10.17 UA_1.7 | CN_6.2 v23.47,13.67 | LC_131.1 v23.3,21.54 | CC_123.2 v22.53,23.02 | CC_124.2 22.53,20.25 v23.14,20.25 | CC_151.2 v26.19,18.9 | v24.46,21.24 CC_141.2 | UY_1.37 14.15,24.65 UY_1.P$10 | UY_1.P$10 UY_1.P$11 | UY_1.36 14.48,25.15 UY_1.P$23 | UY_1.32 14.48,27.15 UY_1.P$23 | UY_1.P$23 12.23,27.65 UY_1.31 | UY_1.23 15.73,26.68 UY_1.P$12 | UY_1.P$20 UY_1.P$23 | UY_1.21 16.73,28.33 | 16.73,27.68 16.41,27.36 UY_1.P$12 | UY_1.P$12 UY_1.P$10 | UY_1.20 16.76,27.65 16.73,27.68 | UY_1.12 16.23,23.65 | UY_1.9 16.23,23.65 | 16.23,23.65 UY_1.P$17 | UY_1.4 13.73,23.89 UY_1.P$3 | UY_1.2 12.73,23.65 | UY_1.39 12.73,23.65 | 12.73,23.65 UY_1.P$4 | UY_1.5 14.23,25.15 UY_1.P$23 | UY_1.14 15.36,24.65 UY_1.P$15 | UY_1.15 14.84,25.15 UY_1.P$13 | UY_1.17 15.21,26.15 UY_1.P$12 | UY_1.18 15.47,26.65 UY_1.P$19 | UR_1.P$2 11.33,16.79 | 10.81,16.53 10.93,16.64 11.18,16.64 11.33,16.79 | UR_1.1 13.07,16.53 12.96,16.64 12.58,16.64 UR_1.P$1 | UR_1.P$5 12.59,17.28 12.59,17.53
  Top 0.229: US_1.7 20.33,17.74 US_1.P$3 | US_1.10 19.86,17.27 US_1.P$3 | US_1.12 19.12,16.26 19.56,16.26 19.84,16.54 US_1.P$2 20.33,16.31 US_1.14 20.33,14.33 | US_1.1 22.73,16.27 22.74,16.26 | US_1.P$4 21.06,17.76 21.34,18.04 21.34,18.49 US_1.5 21.34,18.51 21.34,18.67 | US_1.P$3 19.84,17.51 19.56,17.78 US_1.9 | 16.73,27.68 16.73,28.07 | UA_1.22 12.86,8.39 12.83,8.39 | US_1.7 | CY_351.1 8.51,26.98 v8.05,26.93 | CY_331.1 8.51,27.9 v8.05,27.95 | CY_401.2 v7.8,25.88 | CY_381.1 v7.8,24.86 | v13.23,19.77 13.23,19.95 CY_61.1 | v14.5,19.77 14.5,19.95 CY_71.2 | CY_102.2 16.95,19.54 v16.9,19.49 | UA_1.7 13.46,11.2 CA_9.2 | UA_1.15 11.96,7.77 UA_1.P$2 | CN_181.2 27.94,7.41 UN_1.17 | UN_1.20 29.45,7.26 29.56,7.26 v29.6,7.18 | US_1.7 20.33,19.55
  Top 0.254: IC1.23 47.65,10.89 v47.76,10.97 | UC_1.P$4 27.73,23.91 | UR_1.P$1 12.45,17.02 | IC1.8 43.17,5.48 v42.93,5.59 | IC1.20 46.12,9.39 arc41 45.7,8.97 45.37,8.64 v45.22,8.64 | v23.86,12.27 CN_3.2 | LA_2.2 v18.24,8.03 | CA_16.2 v20.53,7.88 | CA_7.2 v20.53,6.68 | CA_8.2 17.45,6.94 v17.99,7.12 | CA_13.2 v17.94,14.53 | IC1.35 40.17,13.72 39.92,13.97 v39.2,14.61 | CU_3.2 37.34,3.48 v37.04,3.17 | 49.86,12.2 49.86,23.88 49.53,23.88 | v40.64,5.76 40.22,5.34 39.37,5.34 39.17,5.54 39.17,6.15 38.93,6.39 IC1.47 38.14,6.35 | CS_3.2 24.41,19.08 24.41,19.74 | JP6.MTN1 48.45,32.12 | JP6.MTN2 48.45,26.53 v47.74,27.42 | v26.22,26.06 26.29,26.06 | 25.13,7.87 24.52,7.5 | JP6.GND 42.29,26.52
  Top 0.279: IC1.8 43.17,4.31 | IC1.23 45.98,10.89
  Top 0.305: v14.37,14 14.37,14.59 CR_2.2 14.99,14.61 | 15.63,14.99 CR_1.2 15.63,16.39 | 16.73,28.07 16.73,28.33 16.73,28.58 | 16.41,27.36 16.49,27.44 | 27.31,10.55 26.17,11.69 25.79,11.69 25.53,11.94 25.53,14.36 | 27.06,20.83 27.23,21.01 27.23,22.53 | 27.23,22.53 27.56,22.86 27.69,22.86 | 27.23,22.53 26.93,22.23 | 26.93,22.23 26.93,21.9 | 26.93,22.23 26.55,21.85 26.55,21.72 | 11.38,17.76 UR_1.P$3 | CY_31.2 10.97,20.98 v10.97,21.43 | 26.29,26.06 27.92,24.44 | UA_1.22 14.74,6.99 | 28.47,11.9 28.72,12.17 29.05,12.17 29.34,12.45 | US_1.1 21.58,16.27 21.09,16.64
  Top 0.33: UY_1.22 16.23,27.15 | UY_1.19 16.23,27.15 | 16.23,27.15 UY_1.P$20
  Top 1.016: 6.74,15.88 6.74,21.21 6.35,21.59 6.35,23.63 6.61,23.63 6.61,30.36 32.64,30.36 32.64,4.45 6.61,4.45 6.61,10.93 6.23,11.31 6.23,12.96 6.74,13.47 6.74,13.85
  Bottom 0.229: PS1.4 43.2,29.33 43.18,29.34 | 45.22,28.66 45.22,28.96 44.84,28.71
  Bottom 0.254: UY_1.P$12 16.13,26.42 UY_1.P$18 | CU_1.2 39.43,14.1 39.45,13.95 v39.2,14.61 | CU_4.2 43.35,5.08 43.06,5.38 v42.93,5.59 | CU_2.2 46.87,8.65 48.76,8.65 JP3.4 | UN_1.P$1 UN_1.P$9 | 48.65,23.5 49.53,22.74 49.86,22.86 49.86,12.2 47.76,12.2 | RU_1.2 | RU_1.2 v45.22,8.64 | RU_1.2 46.87,8.64 | PS1.1 44.82,27.55 | 39.55,13.97 39.58,13.82
  Bottom 0.305: YN_1.4 28.79,14.19 | YN_1.2 26.21,12.36 26.42,12.83 | YY_1.2 18.51,22.97 v17.84,21.87
  Bottom 0.406: 43.18,29.34 43.18,29.09
  other vias: 19.58,30.32 20.34,20.16 33.23,17.75 27.01,20.8 18.09,12.93 18.24,10.14 10.29,4.48 27.18,27.18 21.54,27.44 19.79,25.91 23.37,26.7 30.13,29.29 6.61,18.67 45.47,14.61 32.6,14.65 34.5,30.79 34.5,27.79 34.5,24.66 32.72,12.22 6.75,4.53 6.62,9.27 7.51,15.66 8.4,19.39 5.27,32.27 2.27,29.27 2.27,24.77 4.76,21.77 1.89,17.14 5.9,15.66 1.89,12.49 5.27,11.27 2.27,9.77 5.27,6.77 2.27,5.27 5.27,2.27 47.75,12.01 32.72,5.97 38.68,31.35 1.89,21.72 3.28,22.86 1.76,19.69 4.81,19.69 3.28,19.69 3.28,16.63 15.39,16.67 15.64,15.02 15.01,14.64 10.43,13.75 37.54,33.43 49.14,32.88 48.5,31.99 47.74,30.98 40.25,33.39 38.47,33.39 49.39,27.42 47.74,25.52 23.8,28.1 26.09,29.88 22.33,30.36 20.34,22.95 17.55,28.54 15.39,30.32 11.2,28.54 11.58,30.32 8.15,30.32 27.54,30.36 25.04,30.82 31.26,30.32 32.66,29.17 32.72,25.96 32.72,23.22 34.5,21.36 18.82,15.84 22.12,15.96 20.68,13.54 21.19,10.62 31.07,18.77 30.31,14.58 23.22,6.3 12.83,4.48 15.88,4.48 18.93,4.48 22.23,4.48 25.4,4.48 28.45,4.48 31.63,4.48 14.31,3.64 10.42,7.14 9.97,32.39 17.67,17.56 17.16,16.04 8.78,22.53 8.78,12.02 6.75,13.5 3.19,13.63 3.22,14.4 6.61,24.52 6.61,27.94 6.61,20.96 3.28,16 7.73,18.66 19,10.39 38.47,26.4 40.63,20.69 40.12,14.09 49.14,24.5 49.14,22.85 38.69,32.49 40.85,26.52 38.44,27.41 40.34,25.5 40.85,24.87 38.44,25.5 39.45,24.36 42.34,27.91 46.42,33 37.79,22.08 49.22,28.68 49.39,25.52 49.39,26.4 41.26,27.55 49.14,30.98 47.74,32.88 49.14,29.71 39.36,33.39 40.58,28.68 39.44,26.4 37.8,24.41 45.72,13.72 40.34,27.46
  pour Bottom (isolate 0.305, rank 2, no thermals): 0.89,1.53 arc65 1.66,0.77 49.1,0.77 arc92 49.99,1.53 49.99,33.02 arc99 49.23,33.81 1.66,33.81 arc100 0.89,33.02
  pour Route2 (isolate 0.305, no thermals): 0.54,34.24 50.24,34.24 50.24,0.54 0.54,0.54
  pour Top: 26.93,10.67 27.18,10.93 28.71,10.93 29.47,10.16 29.47,8.64 29.21,8.39 27.18,8.39 26.93,8.64
  pour Top (isolate 0.305, rank 2, no thermals): 0.89,1.53 arc65 1.66,0.77 49.1,0.77 arc92 49.99,1.53 49.99,33.02 arc99 49.23,33.81 1.66,33.81 arc100 0.89,33.02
